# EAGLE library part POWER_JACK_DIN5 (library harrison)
Digi-Key part number CP-7050-ND
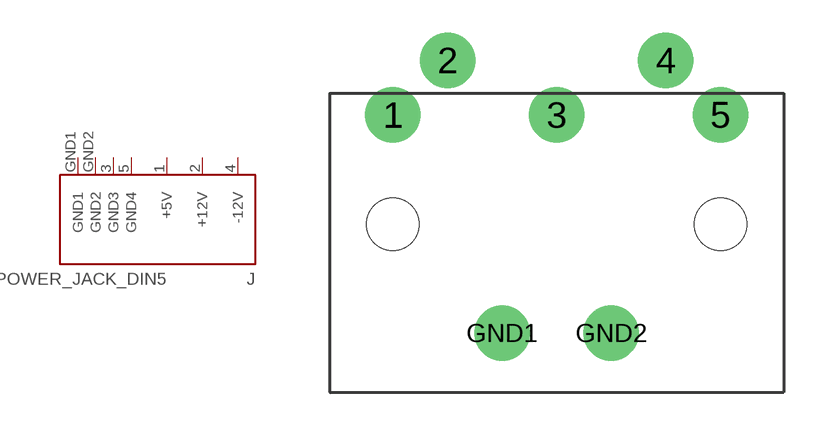
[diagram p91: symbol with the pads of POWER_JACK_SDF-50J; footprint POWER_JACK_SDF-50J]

Designator prefix J

## POWER_JACK_DIN5  [POWER_JACK_SDF-50J]
1  +5V  pwr
2  +12V  pwr
3  GND3  pwr
4  -12V  pwr
5  GND4  pwr
GND1  GND1  pwr
GND2  GND2  pwr

## Footprint POWER_JACK_SDF-50J (pad centres in mm)
Digi-Key part number CP-7050-ND
drill 1.3 pad 2.54: 1 -7.5,5; 2 -5,7.5; 3 0,5; 4 5,7.5; 5 7.5,5; GND1 -2.5,-5; GND2 2.5,-5
hole 2.4 at -7.5,0
hole 2.4 at 7.5,0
